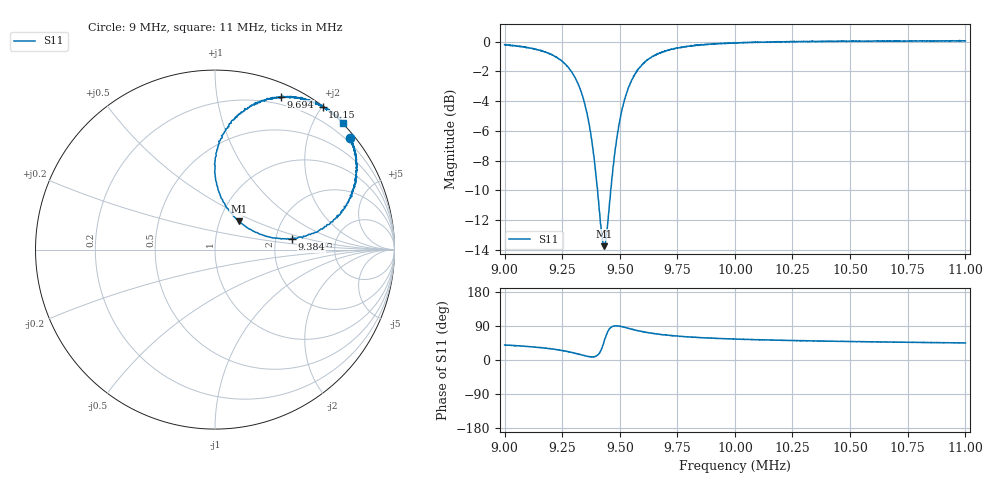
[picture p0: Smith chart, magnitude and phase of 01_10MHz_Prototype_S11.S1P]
! HP8714ET: E.06.02
! Reflection DATA:
# MHz  S  RI  R 50.0
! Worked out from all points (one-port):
!   1601 points, 9 MHz to 11 MHz, reference 50 ohm
!   lowest |S11| = -13.8 dB at 9.433 MHz (marker M1), VSWR 1.52, Z = 61.6 + j20.2 ohm
!   |S11| at or under -10 dB: 9.404 MHz to 9.461 MHz (56.93 kHz wide, 0.604 % of centre)
!   S11 on the Smith chart (normalised r, x): 9 MHz: 0.10, +2.78; 9.384 MHz: 2.47, +0.37; 9.694 MHz: 0.12, +1.52; 10.15 MHz: 0.01, +2.01; 11 MHz: -0.02, +2.43
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9  0.7534 0.6216
9.078  0.7689 0.5758
9.159  0.7851 0.508
9.213  0.7893 0.4287
9.251  0.7758 0.3628
9.293  0.741 0.2687
9.328  0.6727 0.1744
9.358  0.5675 0.0967
9.384  0.4295 0.0602
9.403  0.314 0.0675
9.421  0.1972 0.1132
9.433  0.1323 0.157
9.443  0.0872 0.2075
9.466  0.0144 0.3486
9.481  -0.00106 0.4395
9.501  0.0103 0.5486
9.536  0.0754 0.6915
9.576  0.1651 0.7854
9.621  0.2631 0.8307
9.694  0.3684 0.8509
9.752  0.4285 0.8498
9.86  0.5077 0.8358
10.002  0.5643 0.8125
10.15  0.5996 0.7953
10.252  0.6227 0.7848
10.502  0.6656 0.7509
10.751  0.6877 0.7315
11.001  0.715 0.7067
